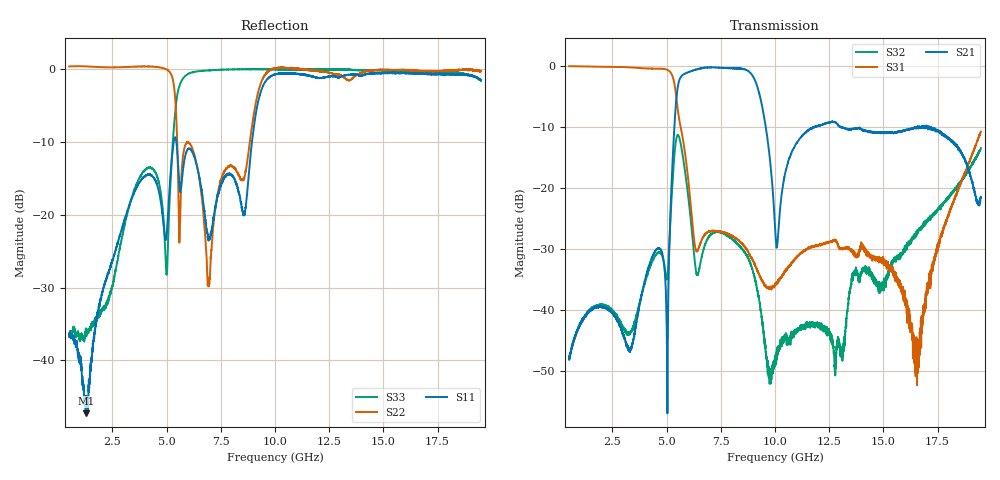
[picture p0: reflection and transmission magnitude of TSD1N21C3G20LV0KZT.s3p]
# MHZ S RI R 50
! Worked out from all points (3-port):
!   3801 points, 500 MHz to 19.5 GHz, reference 50 ohm
!   strongest paths, dB at 500 MHz, 5.25 GHz, 10 GHz, 14.75 GHz, 19.5 GHz:
!     S21: -48.2, -17.5, -26.4, -11.0, -21.5
!     S31: -0.1, -1.5, -35.9, -31.7, -10.8
!     S32: -47.8, -20.3, -47.9, -36.5, -13.5
!   lowest |S11| = -47.3 dB at 1.265 GHz (marker M1), VSWR 1.01, Z = 50 - j0.433 ohm
!   |S11| at or under -10 dB: start of sweep to 5.325 GHz; 5.448 GHz to 8.936 GHz (3.488 GHz wide, 48.5 % of centre)
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500  0.0139 0.00514  0.000544 0.00394  0.9676 -0.212
     0.000482 0.00388  1.029 -0.1426  0.000662 0.00388
     0.9679 -0.211  0.000958 0.00396  0.0134 0.00679
1265  0.000309 -0.00432  0.0032 0.0084  0.8481 -0.5019
      0.00323 0.00848  0.9703 -0.3788  0.00474 0.00788
      0.8483 -0.5017  0.0048 0.00769  0.0133 -0.00709
5010  0.0734 -0.0168  -0.00457 -0.00319  -0.9263 -0.0448
      -0.00464 -0.00337  -0.45 -0.8801  -0.00324 0.0174
      -0.9268 -0.0446  -0.00308 0.0174  -0.0367 -0.0138
5270  0.2695 -0.0392  0.1576 -0.0156  -0.6974 0.4308
      0.158 -0.0156  -0.7884 -0.3518  -0.0692 0.0858
      -0.6987 0.4323  -0.0693 0.0857  -0.0546 0.2874
5645  0.1071 -0.0964  -0.3203 -0.738  -0.1089 0.2967
      -0.3202 -0.7382  0.083 -0.105  0.2312 -0.0187
      -0.1089 0.2958  0.2306 -0.0186  0.7 0.3958
6945  0.0453 -0.049  -0.3598 0.8988  -0.0436 -0.0048
      -0.361 0.8981  0.00359 0.033  0.0289 0.0271
      -0.0434 -0.00514  0.0291 0.0271  0.4653 -0.8607
8675  -0.1224 0.0135  0.9009 0.2137  -0.0261 0.0175
      0.8987 0.2134  0.204 0.051  0.0192 -0.0206
      -0.0259 0.0178  0.019 -0.0207  -0.0444 -0.9935
10000  0.9185 0.0212  0.0305 -0.0374  0.0126 0.00952
       0.0303 -0.0372  0.9412 -0.3664  0.00379 0.000504
       0.0126 0.00985  0.00395 0.000801  -0.3198 -0.9381
16545  -0.4859 -0.7935  0.2866 -0.1041  -0.00362 -0.00278
       0.2872 -0.1061  -0.1799 -0.9533  -0.0221 0.0346
       -0.00287 -0.00206  -0.0211 0.0362  -0.9499 0.0977
19500  -0.7966 0.2299  0.0819 0.0175  0.1919 0.2133
       0.0825 0.0165  -0.8431 -0.468  0.0712 0.1996
       0.1965 0.211  0.0716 0.1986  -0.5598 0.6187
